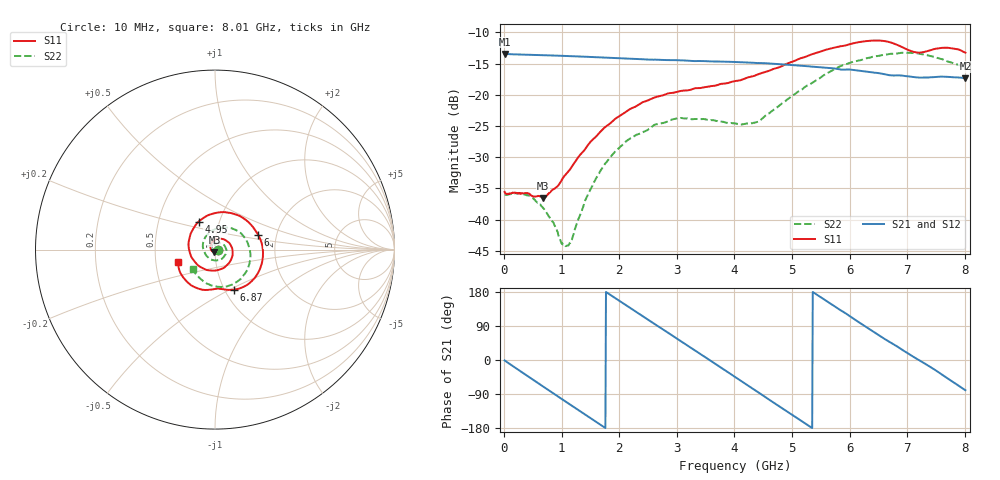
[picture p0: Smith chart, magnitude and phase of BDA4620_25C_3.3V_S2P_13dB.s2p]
!Agilent Technologies,E5071B,MY42404982,A.09.10
!Date: Wed May 06 08:51:17 2026
!Data & Calibration Information:
!Freq	S11:SOLT2(ON)	S21:SOLT2(ON)	S12:SOLT2(ON)	S22:SOLT2(ON)
# Hz S RI R 50
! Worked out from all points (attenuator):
!   801 points, 10 MHz to 8.01 GHz, reference 50 ohm
!   highest |S21| = -13.43 dB at 10 MHz (marker M1); lowest = -17.4 dB at 8.01 GHz (marker M2)
!   lowest |S11| = -36.5 dB at 680 MHz (marker M3), VSWR 1.03, Z = 49.7 - j1.45 ohm
!   |S11| at or under -10 dB: start of sweep to end of sweep
!   |S22| runs from -44.3 to -13.2 dB; largest |S21 - S12| = 0.00097
!   S11 on the Smith chart (normalised r, x): 10 MHz: 1.03, -0.00; 4.95 GHz: 0.80, +0.26; 6 GHz: 1.60, +0.28; 6.87 GHz: 1.10, -0.52; 8.01 GHz: 0.65, -0.10
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1e7  0.0166 -0.0012  0.213 -0.0046  0.2134 -0.00467  0.0159 -0.000704
4.2e8  0.0092 -0.0133  0.1521 -0.1444  0.1523 -0.1446  0.0138 -0.00715
6.8e8  -0.00311 -0.0146  0.071 -0.1955  0.071 -0.1959  0.00771 -0.00966
1.08e9  -0.0232 0.00132  -0.0729 -0.1915  -0.073 -0.1919  -0.00497 -0.00358
1.16e9  -0.0246 0.00773  -0.0989 -0.1787  -0.0992 -0.1789  -0.00668 -0.000545
1.35e9  -0.0247 0.0236  -0.1512 -0.135  -0.1514 -0.1352  -0.00885 0.00766
1.59e9  -0.0136 0.0439  -0.1913 -0.0606  -0.1915 -0.0606  -0.00657 0.02
1.9e9  0.0171 0.06  -0.1923 0.0467  -0.1926 0.0469  0.00648 0.0332
2.31e9  0.0672 0.0467  -0.1116 0.1588  -0.1118 0.1589  0.034 0.0339
2.68e9  0.0972 -0.000402  0.00515 0.191  0.00535 0.1913  0.0556 0.0176
3.4e9  0.0342 -0.1079  0.1787 0.0536  0.179 0.0535  0.0453 -0.045
4.01e9  -0.0956 -0.0864  0.1305 -0.1288  0.1305 -0.1291  -0.0245 -0.0537
4.41e9  -0.1459 0.00687  0.0159 -0.179  0.0158 -0.1796  -0.06 -0.00991
4.95e9  -0.0914 0.1556  -0.1323 -0.113  -0.1326 -0.1133  -0.0427 0.0837
5.35e9  0.0364 0.2089  -0.1683 -0.0013  -0.1684 -0.00114  0.031 0.1207
6e9  0.241 0.0822  -0.0698 0.1434  -0.07 0.1437  0.1697 0.0608
6.34e9  0.2633 -0.0649  0.0216 0.151  0.0219 0.1511  0.197 -0.0231
6.68e9  0.1782 -0.197  0.0947 0.1084  0.0951 0.1086  0.1777 -0.1157
6.87e9  0.1031 -0.2238  0.1223 0.0744  0.1226 0.0745  0.1463 -0.1592
7.18e9  0.0169 -0.2175  0.1377 0.0046  0.138 0.00459  0.0644 -0.205
7.56e9  -0.096 -0.2163  0.1161 -0.0782  0.1165 -0.0783  -0.0402 -0.1911
8.01e9  -0.2059 -0.071  0.024 -0.1334  0.0243 -0.1336  -0.1235 -0.1106
